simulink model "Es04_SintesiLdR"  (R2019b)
settings: Solver=ode4  StartTime=0.0  StopTime=15  FixedStep=0.0001  RelTol=1e-3
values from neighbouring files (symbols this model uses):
  Tc = 1    [Es04_svolgimento.m]
undefined symbols (not defined in the file or in its folder): denP, k, numP

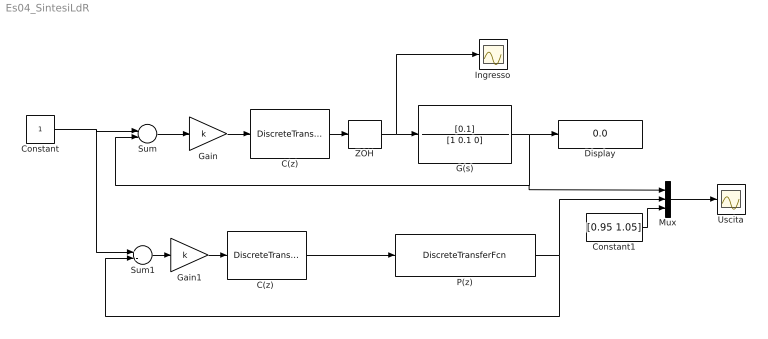
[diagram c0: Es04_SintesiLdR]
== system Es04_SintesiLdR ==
  C(z) : DiscreteTransferFcn  Numerator="[1   -0.9048]"  Denominator=[1 -0.1]  SampleTime=Tc
  "C(z) " : DiscreteTransferFcn  Numerator="[1   -0.9048]"  Denominator=[1 -0.1]  SampleTime=Tc
  Constant : Constant
  Constant1 : Constant  Value=[0.95 1.05]
  Display : Display
  G(s) : TransferFcn  Numerator=[0.1]  Denominator=[1 0.1 0]
  Gain : Gain  Gain=k
  Gain1 : Gain  Gain=k
  Ingresso : Scope
  Mux : Mux  Inputs=3
  P(z) : DiscreteTransferFcn  Numerator=numP  Denominator=denP  SampleTime=Tc
  Sum : Sum  Inputs=+-
  Sum1 : Sum  Inputs=+-
  Uscita : Scope
  ZOH : ZeroOrderHold  SampleTime=Tc
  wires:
  ZOH/1 -> Ingresso/1, G(s)/1
  Sum/1 -> Gain/1
  G(s)/1 -> Display/1, Mux/1, Sum/2
  P(z)/1 -> Sum1/2, Mux/2
  Sum1/1 -> Gain1/1
  Constant/1 -> Sum1/1, Sum/1
  Mux/1 -> Uscita/1
  Gain/1 -> C(z)/1
  C(z)/1 -> ZOH/1
  Gain1/1 -> "C(z) "/1
  "C(z) "/1 -> P(z)/1
  Constant1/1 -> Mux/3
